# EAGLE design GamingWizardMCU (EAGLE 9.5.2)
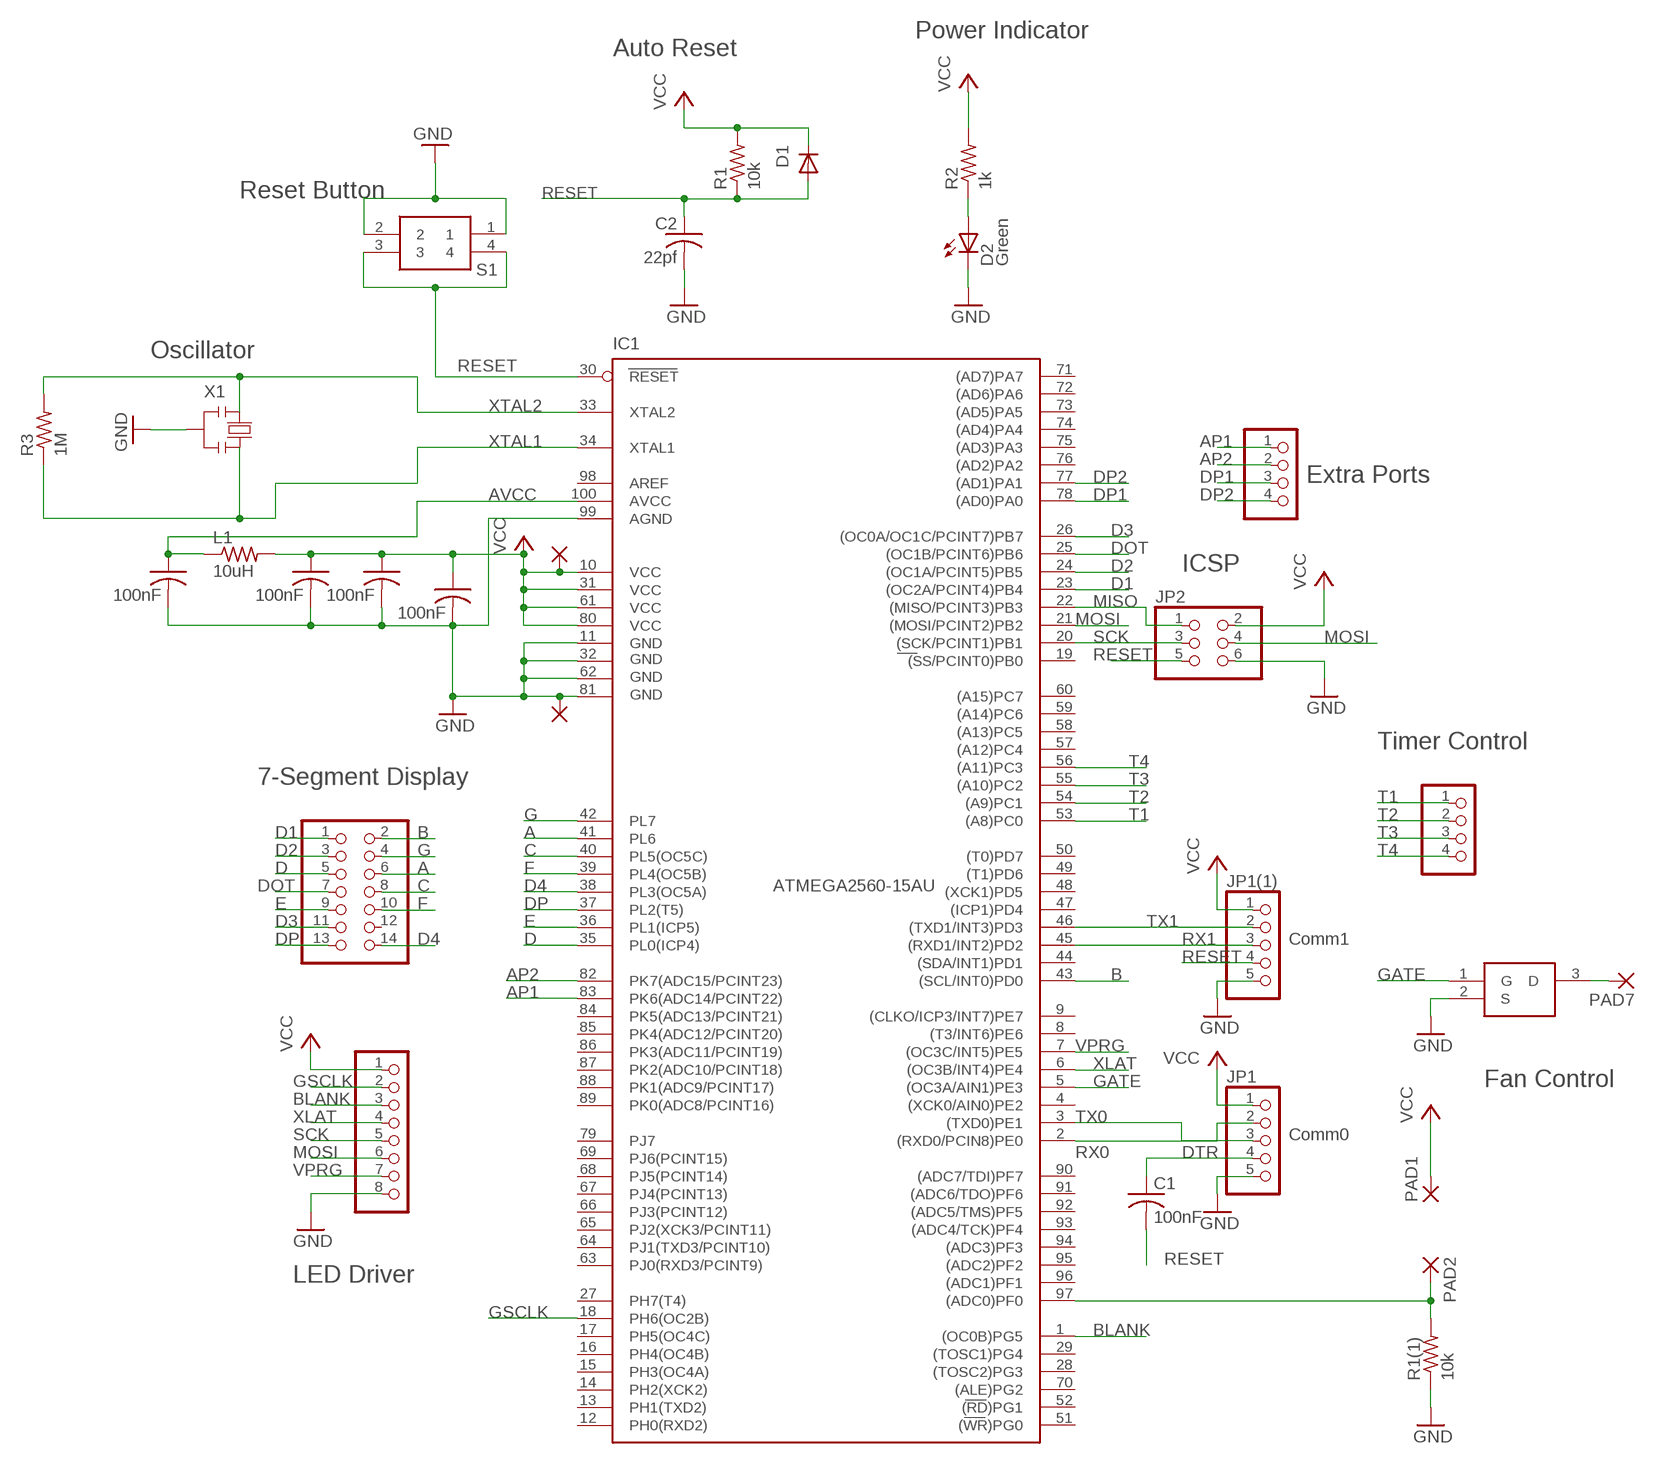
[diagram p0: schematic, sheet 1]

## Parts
C  100nF  C-USC0805  [C0805]
C1  100nF  C-USC0805  [C0805]
C2  22pf  C-USC0805  [C0805]
C3  100nF  C-USC0805  [C0805]
C7  100nF  C-USC0805  [C0805]
C9  100nF  C-USC0805  [C0805]
D1  CD1206-S01575  0012_CD1206-S01575  [MINIMELF]
D2  Green  0043_KPT-2012SGC  [CHIPLED_0805]
IC1  ATMEGA2560-15AU  0023_ATMEGA2560-16AU  [TQFP100]
JP1  PINHD-1X5  [1X05]
JP1(1)  PINHD-1X5  [1X05]
JP2  0114_PH254-203DF118A00V  [2X03]
JP4  PINHD-2X7  [2X07]
JP5  PINHD-1X4  [1X04]
JP6  PINHD-1X8  [1X08]
JP7  PINHD-1X4  [1X04]
L1  10uH  R-US_R0805  [R0805]
PAD1  1,6/0,8  [1,6/0,8]
PAD2  1,6/0,8  [1,6/0,8]
PAD7  1,6/0,8  [1,6/0,8]
PAD8  1,6/0,8  [1,6/0,8]
PAD9  1,6/0,8  [1,6/0,8]
Q1  FDN359BN  [SOT95P251X112-3N]
R1  10k  R-US_R0805  [R0805]
R1(1)  10k  R-US_R0805  [R0805]
R2  1k  R-US_R0805  [R0805]
R3  1M  R-US_R0805  [R0805]
S1  PTS647SN50SMTR2LFS  [PTS647SN50SMTR2LFS]
X1  CSTCE16M0V53-R0  0011_CSTCE16M0V53-R0  [RESONATOR]

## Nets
A: IC1.41(PL6) JP4.6
AP1: IC1.83(PK6(ADC14/PCINT22)) JP7.1
AP2: IC1.82(PK7(ADC15/PCINT23)) JP7.2
AVCC: C9.1 IC1.100(AVCC) L1.1
B: IC1.43((SCL/INT0)PD0) JP4.2
BLANK: IC1.1((OC0B)PG5) JP6.3
C: IC1.40(PL5(OC5C)) JP4.8
D: IC1.35(PL0(ICP4)) JP4.5
D1: IC1.23((OC2A/PCINT4)PB4) JP4.1
D2: IC1.24((OC1A/PCINT5)PB5) JP4.3
D3: IC1.26((OC0A/OC1C/PCINT7)PB7) JP4.11
D4: IC1.38(PL3(OC5A)) JP4.14
DOT: IC1.25((OC1B/PCINT6)PB6) JP4.7
DP: IC1.37(PL2(T5)) JP4.13
DP1: IC1.78((AD0)PA0) JP7.3
DP2: IC1.77((AD1)PA1) JP7.4
DTR: C1.1 JP1.4
E: IC1.36(PL1(ICP5)) JP4.9
F: IC1.39(PL4(OC5B)) JP4.10
FAN: PAD7.1(P) Q1.3(D)
G: IC1.42(PL7) JP4.4
GATE: IC1.5((OC3A/AIN1)PE3) Q1.1(G)
GND: C2.2 C3.2 C7.2 C9.2 C.2 D2.C IC1.11(GND) IC1.32(GND1) IC1.62(GND2) IC1.81(GND3) IC1.99(AGND) JP1(1).5 JP1.5 JP2.6 JP6.8 PAD9.1(P) Q1.2(S) R1(1).1 S1.1 S1.2 X1.2
GSCLK: IC1.18(PH6(OC2B)) JP6.2
MISO: IC1.22((MISO/PCINT3)PB3) JP2.1
MOSI: IC1.21((MOSI/PCINT2)PB2) JP2.4 JP6.6
N$3: D2.A R2.1
RESET: C1.2 C2.1 D1.A IC1.30(RESET) JP1(1).4 JP2.5 R1.1 S1.3 S1.4
RX0: IC1.2((RXD0/PCIN8)PE0) JP1.2
RX1: IC1.45((RXD1/INT2)PD2) JP1(1).3
SCK: IC1.20((SCK/PCINT1)PB1) JP2.3 JP6.5
T1: IC1.53((A8)PC0) JP5.1
T2: IC1.54((A9)PC1) JP5.2
T3: IC1.55((A10)PC2) JP5.3
T4: IC1.56((A11)PC3) JP5.4
THERMISTOR: IC1.97((ADC0)PF0) PAD2.1(P) R1(1).2
TX0: IC1.3((TXD0)PE1) JP1.3
TX1: IC1.46((TXD1/INT3)PD3) JP1(1).2
VCC: C3.1 C7.1 C.1 D1.C IC1.10(VCC) IC1.31(VCC1) IC1.61(VCC2) IC1.80(VCC3) JP1(1).1 JP1.1 JP2.2 JP6.1 L1.2 PAD1.1(P) PAD8.1(P) R1.2 R2.2
VPRG: IC1.7((OC3C/INT5)PE5) JP6.7
XLAT: IC1.6((OC3B/INT4)PE4) JP6.4
XTAL1: IC1.34(XTAL1) R3.1 X1.3
XTAL2: IC1.33(XTAL2) R3.2 X1.1
Unconnected: IC1.4((XCK0/AIN0)PE2) IC1.8((T3/INT6)PE6) IC1.9((CLKO/ICP3/INT7)PE7) IC1.12(PH0(RXD2)) IC1.13(PH1(TXD2)) IC1.14(PH2(XCK2)) IC1.15(PH3(OC4A)) IC1.16(PH4(OC4B)) IC1.17(PH5(OC4C)) IC1.19((SS/PCINT0)PB0) IC1.27(PH7(T4)) IC1.28((TOSC2)PG3) IC1.29((TOSC1)PG4) IC1.44((SDA/INT1)PD1) IC1.47((ICP1)PD4) IC1.48((XCK1)PD5) IC1.49((T1)PD6) IC1.50((T0)PD7) IC1.51((WR)PG0) IC1.52((RD)PG1) IC1.57((A12)PC4) IC1.58((A13)PC5) IC1.59((A14)PC6) IC1.60((A15)PC7) IC1.63(PJ0(RXD3/PCINT9)) IC1.64(PJ1(TXD3/PCINT10)) IC1.65(PJ2(XCK3/PCINT11)) IC1.66(PJ3(PCINT12)) IC1.67(PJ4(PCINT13)) IC1.68(PJ5(PCINT14)) IC1.69(PJ6(PCINT15)) IC1.70((ALE)PG2) IC1.71((AD7)PA7) IC1.72((AD6)PA6) IC1.73((AD5)PA5) IC1.74((AD4)PA4) IC1.75((AD3)PA3) IC1.76((AD2)PA2) IC1.79(PJ7) IC1.84(PK5(ADC13/PCINT21)) IC1.85(PK4(ADC12/PCINT20)) IC1.86(PK3(ADC11/PCINT19)) IC1.87(PK2(ADC10/PCINT18)) IC1.88(PK1(ADC9/PCINT17)) IC1.89(PK0(ADC8/PCINT16)) IC1.90((ADC7/TDI)PF7) IC1.91((ADC6/TDO)PF6) IC1.92((ADC5/TMS)PF5) IC1.93((ADC4/TCK)PF4) IC1.94((ADC3)PF3) IC1.95((ADC2)PF2) IC1.96((ADC1)PF1) IC1.98(AREF) JP4.12

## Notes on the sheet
- Power Indicator
- Auto Reset
- Reset Button
- Oscillator
- Extra Ports
- ICSP
- Timer Control
- 7-Segment Display
- Comm1
- Fan Control
- Comm0
- LED Driver

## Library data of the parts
C C1 C3 C7 C9 = rcl:C-US: CAPACITOR, American symbol; MANUFACTURER: Samsung Electro-Mechanics; MANUFACTURER_PART_NUMBER: CL21F104ZBCNNNC; SPICEPREFIX: C
C2 = rcl:C-US: CAPACITOR, American symbol; MANUFACTURER: FH(Guangdong Fenghua Advanced Tech); MANUFACTURER_PART_NUMBER: 0805CG220J500NT; SPICEPREFIX: C
D1 = Diodi:0012_CD1206-S01575: small-signal high-speed Switching Diodes CD1206; CASE: 1206; MANUFACTURER: Bourns; MANUFACTURER_PART_NUMBER: CD1206-S01575; MONTHLY_USAGE: _____; PART_NUMBER: CD1206-S01575; PRICE: _____; SUPPLIER: _____; TYPE: Diodi
D2 = Opto:0043_KPT-2012SGC: LED GREEN - SMD-0805; MANUFACTURER: Foshan NationStar Optoelectronics; MANUFACTURER_PART_NUMBER: NCD0805G1; MONTHLY_USAGE: _____; PRICE: _____; SUPPLIER: _____; TYPE: Opto
IC1 = IntegratedCircuits:0023_ATMEGA2560-16AU: 8-bit Microcontroller with 256K Bytes In-System Programmable Flash - ATMEGA2560-16AU; CASE: TQFP100_14x14; MONTHLY_USAGE: _____; PART_NUMBER: ATMEGA2560-16AU; PRICE: _____; SUPPLIER: _____; TYPE: Circuito_Integrato
JP1 JP1(1) = pinhead:PINHD-1X5: PIN HEADER; MANUFACTURER: BOOMELE(Boom Precision Elec); MANUFACTURER_PART_NUMBER: C50950
JP2 = Connettori:0114_PH254-203DF118A00V: 3x2 M V h 8,5 mm p2,54; MANUFACTURER: MINTRON; MANUFACTURER_PART_NUMBER: MTP125-1203S1; MONTHLY_USAGE: _____; PART_NUMBER: PH254-203DF118A00V; PRICE: _____; SUPPLIER: _____; TYPE: Connettori; VALUE: ICSP
JP4 = pinhead:PINHD-2X7: PIN HEADER
JP5 JP7 = pinhead:PINHD-1X4: PIN HEADER
JP6 = pinhead:PINHD-1X8: PIN HEADER
L1 = rcl:R-US_: RESISTOR, American symbol; MANUFACTURER: FH(Guangdong Fenghua Advanced Tech); MANUFACTURER_PART_NUMBER: CMI201209X100KT; SPICEPREFIX: R
PAD1 PAD2 PAD7-PAD9 = wirepad:1,6/0,8: THROUGH-HOLE PAD
Q1 = FDN359NSOT:FDN359BN: FDN359BN, N-channel MOSFET Transistor 2.7 A 30 V, 3-Pin SuperSOT Source: Datasheet; DESCRIPTION: FDN359BN, N-channel MOSFET Transistor 2.7 A 30 V, 3-Pin SuperSOT; HEIGHT: 1.12mm; MANUFACTURER_NAME: ON Semiconductor; MANUFACTURER_PART_NUMBER: FDN359BN; MOUSER_PART_NUMBER: 512-FDN359BN; MOUSER_PRICE-STOCK: https://www.mouser.com/Search/Refine.aspx?Keyword=512-FDN359BN
R1 R1(1) = rcl:R-US_: RESISTOR, American symbol; MANUFACTURER: UNI-ROYAL(Uniroyal Elec); MANUFACTURER_PART_NUMBER: 0805W8F1002T5E; SPICEPREFIX: R
R2 = rcl:R-US_: RESISTOR, American symbol; MANUFACTURER: UNI-ROYAL(Uniroyal Elec); MANUFACTURER_PART_NUMBER: 0805W8F1001T5E; SPICEPREFIX: R
R3 = rcl:R-US_: RESISTOR, American symbol; MANUFACTURER: UNI-ROYAL(Uniroyal Elec); MANUFACTURER_PART_NUMBER: 0805W8F1004T5E; SPICEPREFIX: R
S1 = SamacSys_Parts:PTS647SN50SMTR2LFS: Tactile Switches 50mA 12VDC, 1.0N 5.0mm H, G leads Source: Datasheet; DESCRIPTION: SPST-NO 50mA @ 12VDC Top Actuated Standard SMD Tactile Switches RoHS; MANUFACTURER_NAME: Korean Hroparts Elec; MANUFACTURER_PART_NUMBER: K2-1109SP-A4SA-04
X1 = Cristalli:0011_CSTCE16M0V53-R0: 16Mhz - SMD; MANUFACTURER: Murata Electronics; MANUFACTURER_PART_NUMBER: CSTCE16M0V53-R0; MONTHLY_USAGE: _____; PART_NUMBER: CSTCE16M0V53-R0; PRICE: _____; SUPPLIER: _____; TYPE: Cristalli

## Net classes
0 default: width 0.254 mm, drill 0.406 mm, clearance 0.203 mm

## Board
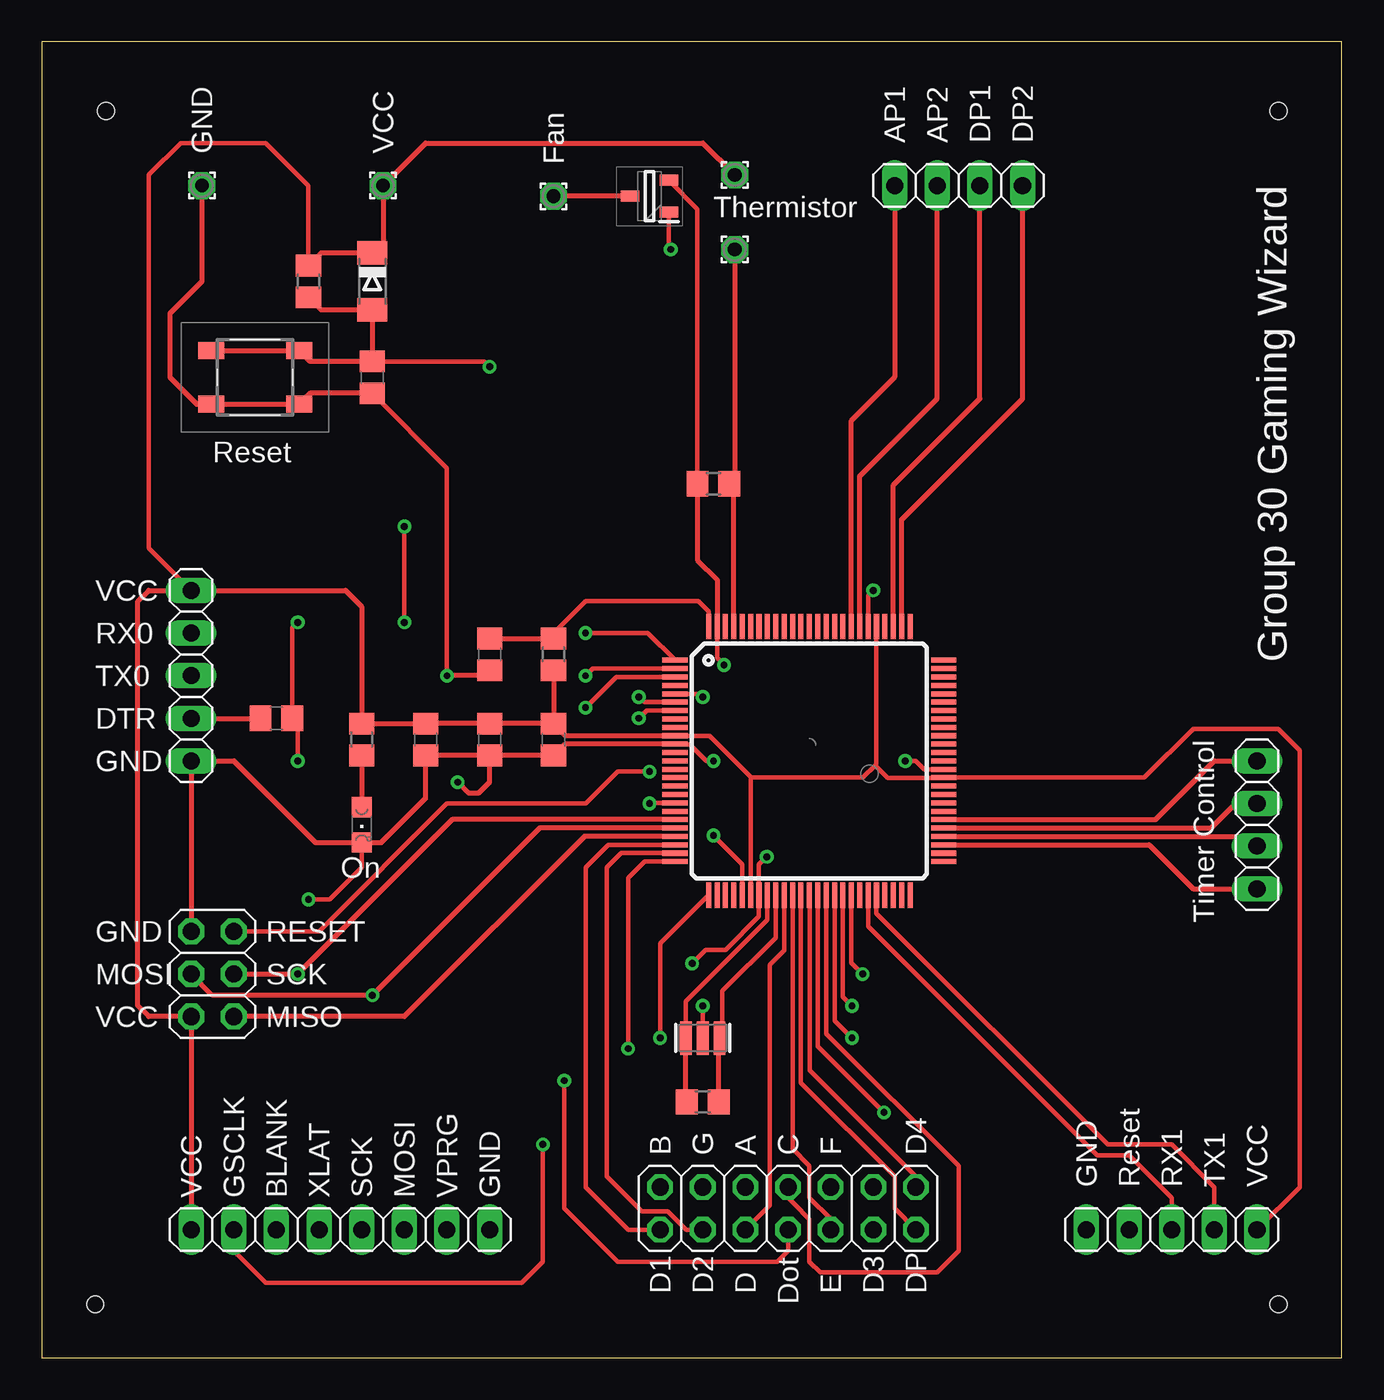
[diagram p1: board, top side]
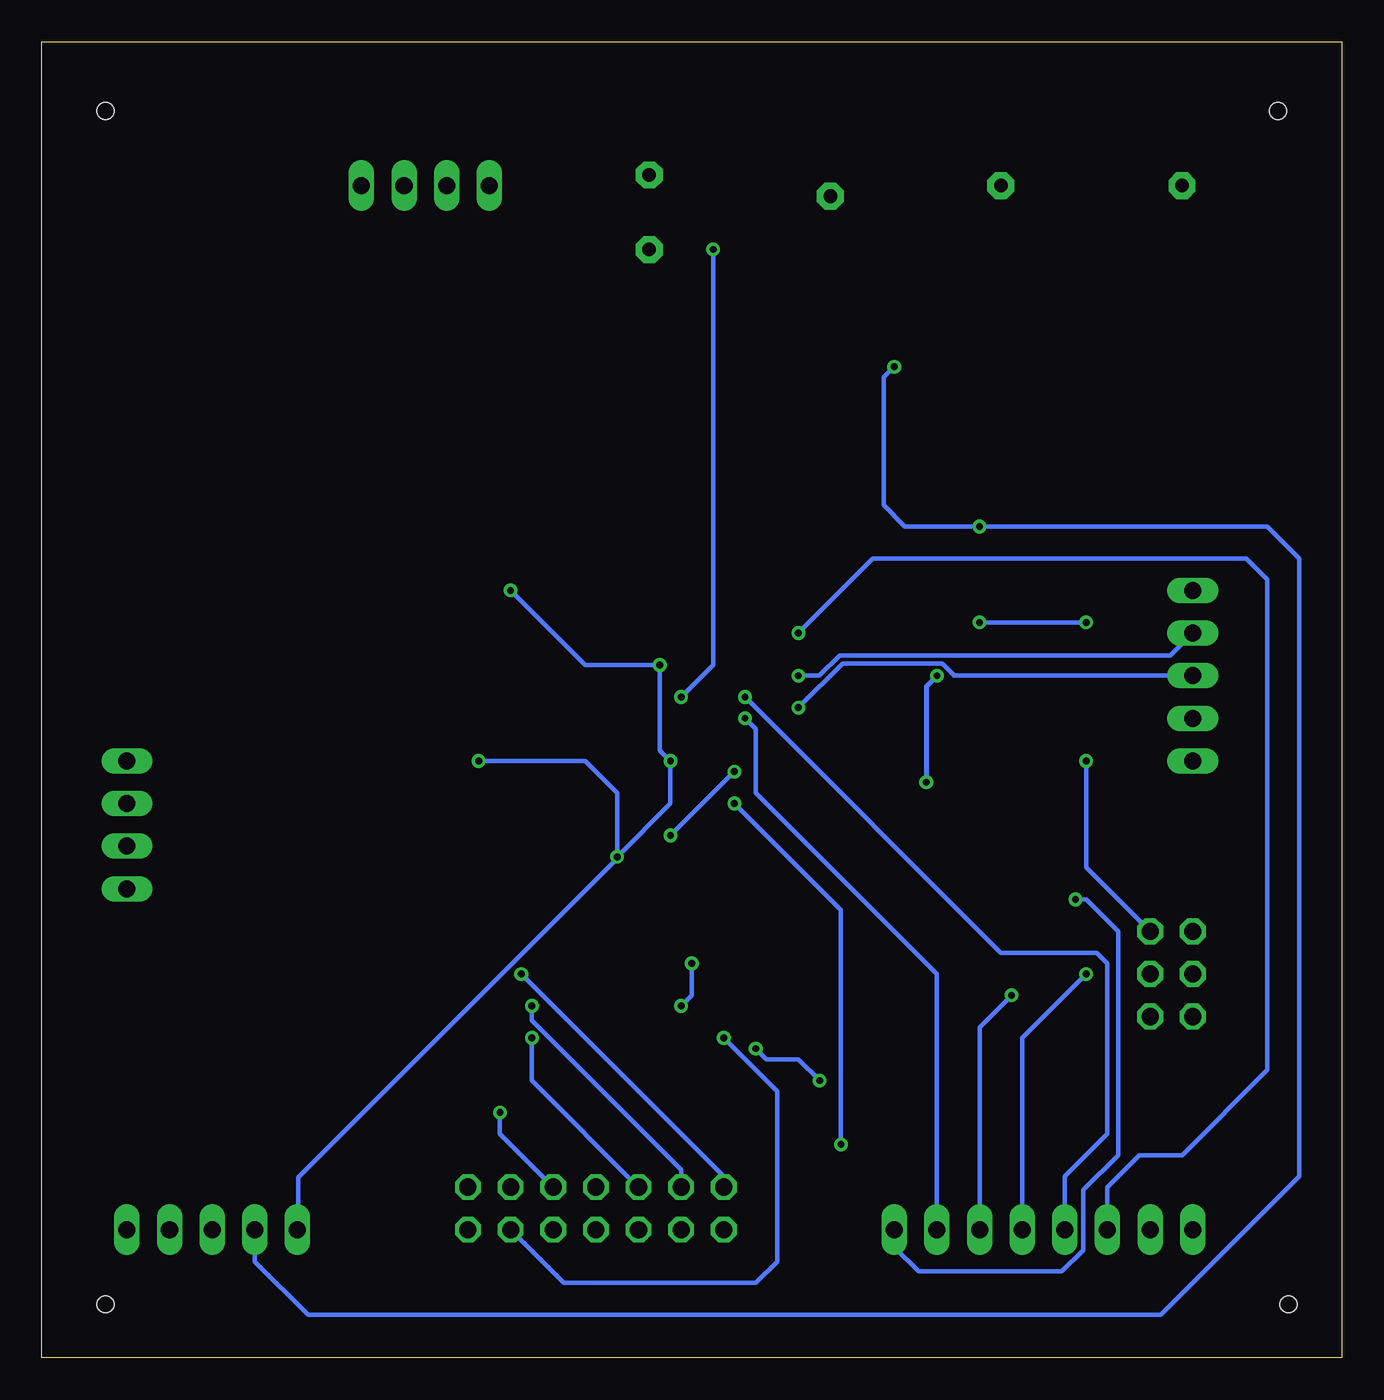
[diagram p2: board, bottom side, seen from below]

Size 77.45 x 78.41 mm. Coordinates in mm from the lower left corner, seen from the top.
Outline: 0,0 77.45,0 77.45,78.41 0,78.41 0,0
Copper layers (1*16): Top 0.035mm / dielectric 1.5mm / Bottom 0.035mm
Design rules "default": minimum track width 6mil, minimum drill 0.35mm, track to track 6mil, track to pad 6mil, pad to pad 6mil, via to via 6mil, smd to smd 6mil, copper to edge 40mil, drill to drill 6mil, minimum pad ring 10mil, minimum via ring 8mil, stop-mask expansion 4mil, vias tented up to drill 0mil, thermal gap 10mil
Holes 1 mm at 3.17,3.17 3.81,74.3 73.66,74.3 73.66,3.17

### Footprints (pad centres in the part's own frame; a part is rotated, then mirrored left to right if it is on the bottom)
C0805 = smd 1.3 x 1.5: 1 -0.95,0; 2 0.95,0
MINIMELF = smd 1.4 x 1.8: A 1.7,0; C -1.7,0
CHIPLED_0805 = smd 1.2 x 1.2: A 0,-1.05; C 0,1.05
TQFP100 = smd 1.5 x 0.3: 1 -8,6; 2 -8,5.5; 3 -8,5; 4 -8,4.5; 5 -8,4; 6 -8,3.5; 7 -8,3; 8 -8,2.5; 9 -8,2; 10 -8,1.5; 11 -8,1; 12 -8,0.5; 13 -8,0; 14 -8,-0.5; 15 -8,-1; 16 -8,-1.5; 17 -8,-2; 18 -8,-2.5; 19 -8,-3; 20 -8,-3.5; 21 -8,-4; 22 -8,-4.5; 23 -8,-5; 24 -8,-5.5; 25 -8,-6; 51 8,-6; 52 8,-5.5; 53 8,-5; 54 8,-4.5; 55 8,-4; 56 8,-3.5; 57 8,-3; 58 8,-2.5; 59 8,-2; 60 8,-1.5; 61 8,-1; 62 8,-0.5; 63 8,0; 64 8,0.5; 65 8,1; 66 8,1.5; 67 8,2; 68 8,2.5; 69 8,3; 70 8,3.5; 71 8,4; 72 8,4.5; 73 8,5; 74 8,5.5; 75 8,6 | smd 0.3 x 1.5: 26 -6,-8; 27 -5.5,-8; 28 -5,-8; 29 -4.5,-8; 30 -4,-8; 31 -3.5,-8; 32 -3,-8; 33 -2.5,-8; 34 -2,-8; 35 -1.5,-8; 36 -1,-8; 37 -0.5,-8; 38 0,-8; 39 0.5,-8; 40 1,-8; 41 1.5,-8; 42 2,-8; 43 2.5,-8; 44 3,-8; 45 3.5,-8; 46 4,-8; 47 4.5,-8; 48 5,-8; 49 5.5,-8; 50 6,-8; 76 6,8; 77 5.5,8; 78 5,8; 79 4.5,8; 80 4,8; 81 3.5,8; 82 3,8; 83 2.5,8; 84 2,8; 85 1.5,8; 86 1,8; 87 0.5,8; 88 0,8; 89 -0.5,8; 90 -1,8; 91 -1.5,8; 92 -2,8; 93 -2.5,8; 94 -3,8; 95 -3.5,8; 96 -4,8; 97 -4.5,8; 98 -5,8; 99 -5.5,8; 100 -6,8
1X05 = drill 1.016 long: 1 -5.08,0; 2 -2.54,0; 3 0,0; 4 2.54,0; 5 5.08,0
2X03 = drill 1.016 pad 1.55 octagon: 1 -2.54,-1.27; 2 -2.54,1.27; 3 0,-1.27; 4 0,1.27; 5 2.54,-1.27; 6 2.54,1.27
2X07 = drill 1.016 octagon: 1 -7.62,-1.27; 2 -7.62,1.27; 3 -5.08,-1.27; 4 -5.08,1.27; 5 -2.54,-1.27; 6 -2.54,1.27; 7 0,-1.27; 8 0,1.27; 9 2.54,-1.27; 10 2.54,1.27; 11 5.08,-1.27; 12 5.08,1.27; 13 7.62,-1.27; 14 7.62,1.27
1X04 = drill 1.016 long: 1 -3.81,0; 2 -1.27,0; 3 1.27,0; 4 3.81,0
1X08 = drill 1.016 long: 1 -8.89,0; 2 -6.35,0; 3 -3.81,0; 4 -1.27,0; 5 1.27,0; 6 3.81,0; 7 6.35,0; 8 8.89,0
R0805 = smd 1.3 x 1.5: 1 -0.95,0; 2 0.95,0
1,6/0,8 = drill 0.813 pad 1.6 octagon: 1 0,0
SOT95P251X112-3N = smd 1.1 x 0.65: 1 -1.15,0.95; 2 -1.15,-0.95; 3 1.15,0
PTS647SN50SMTR2LFS = smd 1.55 x 1: 1 -2.625,-1.6; 2 2.625,-1.6; 3 2.625,1.6; 4 -2.625,1.6
RESONATOR = smd 0.7 x 2: 1 -1,0; 2 0,0; 3 1,0

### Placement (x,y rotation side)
C  30.48,36.83 270 top
C1  13.97,38.1 0 top
C2  19.68,58.42 270 top
C3  26.67,36.83 270 top
C7  22.86,36.83 270 top
C9  26.67,41.91 270 top
D1  19.68,64.14 270 top
D2  19.05,31.75 180 top
IC1  45.72,35.56 0 top
JP1  8.89,40.64 270 top
JP1(1)  67.31,7.62 180 top
JP2  10.16,22.86 90 top
JP4  44.45,8.89 0 top
JP5  72.39,31.75 90 top
JP6  17.78,7.62 0 top
JP7  54.61,69.85 0 top
L1  30.48,41.91 270 top
PAD1  41.27,70.48 0 top
PAD2  41.27,66.04 0 top
PAD7  30.48,69.22 0 top
PAD8  20.32,69.85 0 top
PAD9  9.53,69.85 0 top
Q1  36.2,69.22 180 top
R1  15.88,64.14 90 top
R1(1)  40.01,52.07 0 top
R2  19.05,36.83 90 top
R3  39.37,15.24 180 top
S1  12.7,58.42 0 top
X1  39.37,19.05 0 top

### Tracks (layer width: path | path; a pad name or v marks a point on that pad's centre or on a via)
A  (via drill 0.41)
  Top 0.254: v48.26,19.05 47.24,20.07 47.24,27.54 IC1.41
  Bottom 0.254: v48.26,19.05 48.26,16.51 JP4.6
AP1
  Top 0.305: JP7.1 50.8,58.42 48.22,55.84 IC1.83
AP2
  Top 0.305: IC1.82 48.72,52.53 53.34,57.15 JP7.2
AVCC
  Top 0.254: IC1.100 39.72,44.16 39.74,44.18 39.74,44.45 39.1,45.09 32.38,45.09 30.48,43.18 L1.1
  Top 0.305: C9.1 L1.1
B  (via drill 0.41)
  Top 0.254: v48.9,22.86 48.22,23.54 IC1.43
  Bottom 0.254: JP4.2 36.83,10.79 v48.9,22.86
BLANK  (via drill 0.41)
  Top 0.254: v32.38,43.18 36.1,43.18 IC1.1
  Bottom 0.254: v32.38,43.18 27.94,47.62 5.71,47.62 4.45,46.35 4.45,17.14 9.53,12.06 12.06,12.06 13.97,10.16 JP6.3
C
  Top 0.254: JP4.8 44.45,9.53 45.26,8.71 45.26,8.7 45.72,8.24 45.72,5.71 46.35,5.08 53.34,5.08 54.61,6.35 54.61,11.43 46.74,19.3 46.74,27.54 IC1.40
D
  Top 0.254: JP4.5 43.36,9.07 43.36,23.4 44.22,24.26 IC1.35
D1
  Top 0.254: JP4.1 34.92,7.62 32.38,10.16 32.38,29.21 33.73,30.56 IC1.23
D2
  Top 0.254: JP4.3 38.38,7.62 37.28,8.71 35.74,8.71 33.66,10.79 33.66,29.21 34.51,30.06 IC1.24
D3  (via drill 0.41)
  Top 0.254: IC1.26 36.83,24.67 v36.83,19.05
  Bottom 0.254: JP4.11 46.35,4.45 34.92,4.45 33.66,5.71 33.66,15.88 v36.83,19.05
D4
  Top 0.254: IC1.38 45.74,27.54 45.74,17.12 52.07,10.79 JP4.14
DOT  (via drill 0.41)
  Top 0.254: JP4.7 44.45,6.35 43.81,5.71 34.29,5.71 31.11,8.89 v31.11,16.51 | IC1.25 35.91,29.56 34.92,28.57 v34.92,18.41
  Bottom 0.254: v31.11,16.51 32.38,17.78 34.29,17.78 v34.92,18.41
DP
  Top 0.254: JP4.13 50.8,8.89 50.8,10.79 45.22,16.38 IC1.37
DP1
  Top 0.305: IC1.78 50.72,51.99 55.88,57.15 JP7.3
DP2
  Top 0.305: IC1.77 51.22,49.95 58.42,57.15 JP7.4
DTR
  Top 0.305: JP1.4 C1.1
E
  Top 0.254: JP4.9 46.99,8.26 45.72,9.53 45.72,11.43 44.72,12.43 IC1.36
F  (via drill 0.41)
  Top 0.254: IC1.39 46.22,18.55 v50.16,14.61
  Bottom 0.254: JP4.10 50.16,13.34 v50.16,14.61
FAN
  Top 0.305: Q1.3 PAD7.1
G  (via drill 0.41)
  Top 0.254: v48.26,20.95 47.72,21.5 IC1.42
  Bottom 0.254: v48.26,20.95 48.26,20.09 39.37,11.2 JP4.4
GATE  (via drill 0.41)
  Top 0.254: IC1.5 39.18,39.56 v39.37,39.37 | v37.47,66.04 37.34,66.16 Q1.1
  Bottom 0.254: v37.47,66.04 37.47,41.27 v39.37,39.37
GND  (via drill 0.41)
  Top 0.254: Q1.2 39.05,68.45 R1(1).1 | v24.13,40.64 24.13,53.02 C2.2 | IC1.81 49.22,45.41 v49.53,45.72 | IC1.99 40.22,41.7 v40.64,41.27 | IC1.11 37.74,36.54 38.61,36.54 39.59,35.56 v40.01,35.56 | v43.18,29.84 42.72,29.39 IC1.32 42.72,26.29 40.73,24.3 39.55,24.3 v38.73,23.5 | IC1.62 52.57,35.06 52.07,35.56 v51.44,35.56 | v15.88,27.3 17.14,27.3 19.05,29.21 D2.C | v39.37,20.95 X1.2
  Top 0.305: IC1.11 31.16,36.56 C.2 C3.2 | C3.2 C7.2 22.86,33.34 20.22,30.7 D2.C 16.29,30.7 11.43,35.56 JP1.5 JP2.6 | R1(1).1 39.05,47.53 40.22,46.37 IC1.99 | C2.2 15.97,57.47 S1.2 S1.1 9.22,56.82 7.62,58.42 7.62,62.23 9.53,64.14 PAD9.1 | C9.2 26.35,40.64 v24.13,40.64 | v24.77,34.29 25.4,33.66 26.04,33.66 26.67,34.29 C3.2
  Bottom 0.254: v43.18,29.84 40.01,33.02 v40.01,35.56 40.64,36.2 v40.64,41.27 45.09,41.27 v49.53,45.72 | v43.18,29.84 43.18,33.66 45.09,35.56 v51.44,35.56 | JP6.8 26.67,6.58 25.22,5.13 16.69,5.13 15.42,6.41 15.42,9.98 13.34,12.06 13.34,25.4 15.24,27.3 v15.88,27.3 | v38.73,23.5 38.73,21.59 v39.37,20.95 | JP1(1).5 62.18,7.77 62.18,10.74 43.2,29.72 v43.18,29.84
  Bottom 0.305: v24.13,40.64 24.77,40.01 v24.77,34.29
GSCLK  (via drill 0.41)
  Top 0.254: IC1.18 36.23,33.06 v36.2,33.02 | v29.84,12.7 29.84,5.71 28.57,4.45 13.34,4.45 11.43,6.35 JP6.2
  Bottom 0.254: v36.2,33.02 29.84,26.67 v29.84,12.7
MISO
  Top 0.305: IC1.22 32.33,31.06 21.59,20.32 JP2.1
MOSI  (via drill 0.41)
  Top 0.305: IC1.21 29.66,31.56 v19.68,21.59 10.16,21.59 JP2.4
  Bottom 0.254: v19.68,21.59 21.59,19.68 JP6.6
N$3
  Top 0.305: R2.1 D2.A
RESET  (via drill 0.41)
  Top 0.254: v15.24,35.56 15.24,37.78 C1.2 14.92,43.49 v15.24,43.81 | JP2.5 16.51,25.4 24.13,33.02 32.38,33.02 34.29,34.92 v36.2,34.92 | v40.01,31.11 41.72,29.4 IC1.30 | v21.59,43.81 v21.59,49.53 | C2.1 26.36,59.37 v26.67,59.05
  Top 0.305: S1.4 S1.3 15.97,59.37 C2.1 D1.A 16.62,62.44 R1.1
  Bottom 0.254: v15.24,35.56 15.24,29.21 JP2.5 | v36.2,34.92 v40.01,31.11 | v15.24,43.81 v21.59,43.81 | v26.67,59.05 27.3,58.42 27.3,50.8 26.04,49.53 v21.59,49.53 4.45,49.53 2.54,47.62 2.54,10.79 10.79,2.54 61.59,2.54 64.77,5.71 JP1(1).4
RX0  (via drill 0.41)
  Top 0.254: v32.38,40.64 32.82,41.08 37.7,41.08 IC1.2
  Bottom 0.254: v32.38,40.64 31.13,40.64 29.93,41.83 10.24,41.83 JP1.2
RX1
  Top 0.254: IC1.45 49.22,25.71 62.87,12.06 64.77,12.06 67.31,9.53 JP1(1).3
SCK  (via drill 0.41)
  Top 0.305: JP2.3 v15.24,22.86 24.44,32.06 IC1.20
  Bottom 0.254: v15.24,22.86 19.05,19.05 JP6.5
T1
  Top 0.305: IC1.53 65.96,30.56 68.58,27.94 JP5.1
T2
  Top 0.305: IC1.54 71.81,31.06 JP5.2
T3
  Top 0.305: IC1.55 69.66,31.56 71.12,33.02 JP5.3
T4
  Top 0.305: IC1.56 66.35,32.06 69.85,35.56 JP5.4
THERMISTOR
  Top 0.305: PAD2.1 41.27,52.39 R1(1).2 41.22,51.8 IC1.97
TX0  (via drill 0.41)
  Top 0.254: v32.38,38.73 34.21,40.56 IC1.3
  Bottom 0.254: JP1.3 23.09,40.64 23.82,41.38 29.74,41.38 v32.38,38.73
TX1
  Top 0.254: IC1.46 49.72,26.48 63.5,12.7 67.31,12.7 69.85,10.16 JP1(1).2
VCC
  Top 0.254: JP1(1).1 74.93,10.16 74.93,36.2 73.66,37.47 68.58,37.47 65.67,34.56 IC1.61 53.59,34.54 50.39,34.54 49.64,35.3 | IC1.31 42.22,34.62 | IC1.10 39.77,37.06 42.22,34.62 | R1.2 15.88,69.85 13.34,72.39 8.26,72.39 6.35,70.48 6.35,48.26 JP1.1 | 42.22,34.62 42.27,34.56 48.9,34.56 49.64,35.3 | IC1.80 49.72,35.38 49.64,35.3
  Top 0.305: IC1.10 31.2,37.06 C.1 | C.1 C3.1 C7.1 R2.2 19.05,44.77 18.09,45.72 JP1.1 6.35,45.72 5.71,45.09 5.71,20.95 6.35,20.32 JP2.2 JP6.1 | L1.2 C.1 | R1.2 16.62,65.83 D1.C 20.32,66.47 PAD8.1 22.86,72.39 39.37,72.39 PAD1.1
VPRG  (via drill 0.41)
  Top 0.254: IC1.7 36.02,38.56 v35.56,38.1
  Bottom 0.254: v35.56,38.1 34.92,37.47 34.92,33.66 24.13,22.86 JP6.7
XLAT  (via drill 0.41)
  Top 0.254: IC1.6 35.87,39.06 v35.56,39.37
  Bottom 0.254: v35.56,39.37 20.32,24.13 14.61,24.13 13.97,23.5 13.97,13.34 16.51,10.79 JP6.4
XTAL1
  Top 0.254: X1.3 40.55,19.23 40.55,21.84 43.72,25.02 IC1.34
  Top 0.305: R3.1 40.32,19 X1.3
XTAL2
  Top 0.254: IC1.33 43.22,26.07 38.37,21.23 X1.1
  Top 0.305: R3.2 38.37,15.29 X1.1

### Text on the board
tPlace: GND | VCC | AP1 | AP2 | DP1 | DP2 | Fan | Group 30 Gaming Wizard | Thermistor | Reset | VCC | RX0 | TX0 | DTR | Timer Control | GND | On | GND | RESET | MOSI | SCK | VCC | MISO | B | G | A | C | F | D4 | VCC | GSCLK | BLANK | XLAT | SCK | MOSI | VPRG | GND | GND | Reset | RX1 | TX1 | VCC | D1 | D2 | D | E | D3 | DP | Dot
